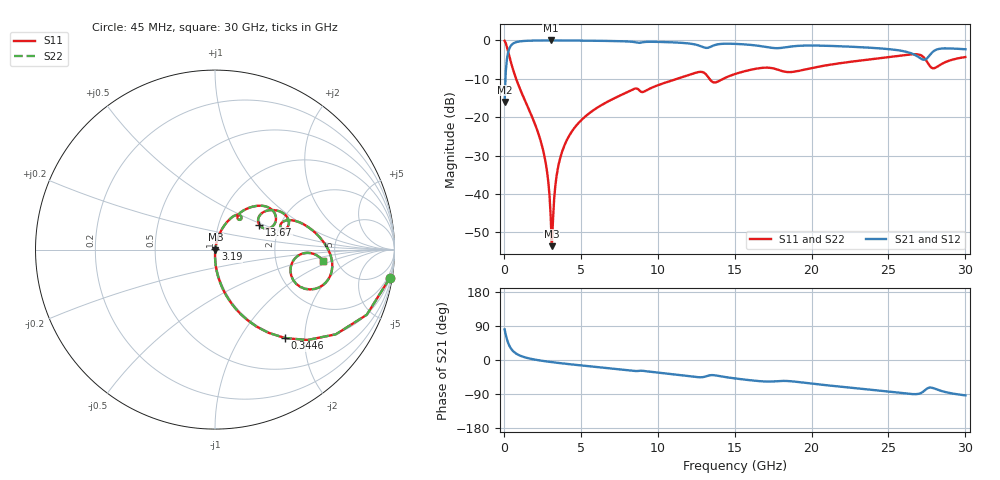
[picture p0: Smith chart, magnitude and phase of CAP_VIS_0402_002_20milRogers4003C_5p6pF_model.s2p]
! S-parameter model data by Modelithics Inc.  support@modelithics.com  813-866-6335  Tampa FL USA
! S-Parameter data specifications:
! Substrate: 20-mil Rogers 4003C, substrate thickness, H=0.508mm, Dielectric constant, Er=3.75
! PCB Mounting Pad Footprint: Pad width, PadW=0.50mm , Pad length, PadL=0.50mm , Pad gap, PadG (edge-to-edge)=0.40mm , Reference planes=1.4mm apart
! Created Wed Nov 18 12:48:32 2015
# hz S ma R 50
! 2 Port Network Data from SP1.SP block
! freq  magS11  angS11  magS21  angS21  magS12  angS12  magS22  angS22
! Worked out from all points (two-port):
!   401 points, 45 MHz to 30 GHz, reference 50 ohm
!   highest |S21| = -0.02 dB at 3.041 GHz (marker M1); lowest = -16.1 dB at 45 MHz (marker M2)
!   |S21| within 3 dB of the highest: 282.6 MHz to 26.2 GHz (25.92 GHz wide, 196 % of centre); 27.88 GHz to end of sweep
!   lowest |S11| = -53.6 dB at 3.115 GHz (marker M3), VSWR 1.00, Z = 50.2 - j0.0467 ohm
!   |S11| at or under -10 dB: 793.1 MHz to 11.27 GHz (10.48 GHz wide, 174 % of centre); 13.36 GHz to 14.26 GHz (903.6 MHz wide, 6.54 % of centre)
!   |S22| runs from -53.6 to -0.1 dB; largest |S21 - S12| = 0
!   S11 on the Smith chart (normalised r, x): 45 MHz: 1, -12; 344.6 MHz: 0.98, -1.61; 3.19 GHz: 1.01, +0.01; 13.67 GHz: 1.57, +0.47; 30 GHz: 3.92, -0.78
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4.5e7  0.9876 -9.1  0.1572 80.9  0.1572 80.9  0.9876 -9.1
3.4455e8  0.6295 -51.6  0.7764 38.4  0.7764 38.4  0.6295 -51.6
8.687625e8  0.2874 -74.7  0.9567 15.1  0.9567 15.1  0.2874 -74.7
2.4414e9  0.04504 -89.5  0.9971 -1.9  0.9971 -1.9  0.04504 -89.5
2.74095e9  0.02372 -88.9  0.9977 -3.6  0.9977 -3.6  0.02372 -88.9
3.0405e9  0.005127 -71.7  0.9978 -5.3  0.9978 -5.3  0.005127 -71.7
3.115388e9  0.002091 -12.8  0.9978 -5.6  0.9978 -5.6  0.002091 -12.8
3.190275e9  0.004582 56.7  0.9978 -6.0  0.9978 -6.0  0.004582 56.7
3.489825e9  0.02064 76.4  0.9975 -7.5  0.9975 -7.5  0.02064 76.4
3.789375e9  0.03588 77.4  0.9969 -8.9  0.9969 -8.9  0.03588 77.4
5.062462e9  0.09279 73.8  0.9928 -14.5  0.9928 -14.5  0.09279 73.8
8.282625e9  0.2252 58.8  0.9614 -28.0  0.9614 -28.0  0.2252 58.8
1.007992e10  0.2638 54.5  0.9554 -33.6  0.9554 -33.6  0.2638 54.5
1.270099e10  0.3882 34.1  0.8538 -45.5  0.8538 -45.5  0.3882 34.1
1.367452e10  0.283 29.2  0.8645 -40.2  0.8645 -40.2  0.283 29.2
1.50225e10  0.3647 36.6  0.901 -48.6  0.901 -48.6  0.3647 36.6
2.003996e10  0.4376 22.0  0.8569 -62.4  0.8569 -62.4  0.4376 22.0
2.505742e10  0.6064 4.0  0.7677 -83.5  0.7677 -83.5  0.6064 4.0
2.670495e10  0.661 -9.6  0.6485 -90.2  0.6485 -90.2  0.661 -9.6
2.737894e10  0.5745 -22.7  0.561 -79.5  0.561 -79.5  0.5745 -22.7
2.835248e10  0.4787 -3.1  0.7794 -80.6  0.7794 -80.6  0.4787 -3.1
3e10  0.6066 -6.0  0.7666 -93.4  0.7666 -93.4  0.6066 -6.0
